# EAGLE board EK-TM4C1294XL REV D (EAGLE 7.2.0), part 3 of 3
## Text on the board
Bottom: EK-TM4C1294XL / REV D
tPlace: DEBUG | TXD | RXD | Target USB | TCK | TMS | TDI | BoosterPack 2 | TDO | BoosterPack 1 | !RESET | TM | Tiva C Series / Connected LaunchPad | 85 | 71 | 57 | 43 | 29 | 15 | 1
bPlace: TXD | RXD | TCK | TMS | TDI | TDO | !RESET
tNames: POWER | http://www.ti.com/launchpad | POWER SELECT | U22 | BoosterPack | +3v3 | OTG | ICDI | U14 | CAN | UART | MCU 3V3 | Y2 | CAN | Y1 | UART | EK-TM4C1294XL Rev D
bNames: +3v3 / PD2 / PP0 / PP1 / See JP4 / See JP5 / PQ0 / PP4 / PN5 / PN4 | +5V / GND / PB4 / PB5 / PK0 / PK1 / PK2 / PK3 / PA4 / PA5 | TP1 | TP8 | +3V3 / PE4 / PC4 / PC5 / PC6 / PE5 / PD3 / PC7 / PB2 / PB3 | TP10 | TP13 | TP3 | +5V / GND / PE0 / PE1 / PE2 / PE3 / PD7 / PA6 / PM4 / PM5 | TP9 | BP2_A2.6 / PA1 | PD5 / ICDI_TX | TP4 | TP5 | PG1 / PK4 / PK5 / PM0 / PM1 / PM2 / PH0 / PH1 / PK6 / PK7 | TP12 | BP2_A2.5 / PA0 | PD4 / ICDI RX | TP2 | TP6 | TP11 | PF1 / PF2 / PF3 / PG0 / PL4 / PL5 / PL0 / PL1 / PL2 / PL3 | TP7 | GND / PM7 / PP5 / PA7 / !RESET / PQ2/PA3 / PQ3/PA2 / PP3 / PQ1 / PM6 | GND / PM3 / PH2 / PH3 / !RST / PD1 / PD0 / PN2 / PN3 / PP2 | 5V / 3V3 | !WAK / GND | PQ4 / !RST | PN3 / PM4 | PN2 / PM5 | PN1 / PM6 | PN0 / PM7 | PN5 / PJ1 | PN4 / PJ0 | PL5 / PP5 | PK4 / PP4 | PK5 / PA1 | PP3 / PA0 | PP2 / PF3 | PB3 / PF2 | PB2 / PF1 | PL4 / PF0 | PK6 / PF4 | GND / GND | PK7 / PB1 | PQ3 / PB0 | PQ2 / PP1 | PQ1 / PP0 | PQ0 / PD2 | PL3 / PD0 | PL2 / PD1 | PL1 / PD3 | PL0 / PD6 | PM0 / PD7 | PM1 / PD4 | PM2 / PD5 | GND / GND | PM3 / REF | PG0 / PK3 | PG1 / PK2 | PA7 / PK1 | PA6 / PK0 | PC4 / PE5 | PC5 / PE4 | PC6 / PE3 | PC7 / PE2 | PH3 / PE1 | PH2 / PE0 | PH1 / PA5 | PH0 / PA4 | PB5 / PA3 | PB4 / PA2 | GND / GND | 3V3 / 5V
Document: Layer Stackup / Top silkscreen / Top Solder Mask / Component Side / Layer 2 / Layer 3 / Solder Side / Bottom Solder Mask / Bottom Silkscreen | File Names / EK-TM4C129EXL.sst / EK-TM4C129EXL.smt / EK-TM4C129EXL.l1 / EK-TM4C129EXL.l2 / EK-TM4C129EXL.l3 / EK-TM4C129EXL.l4 / EK-TM4C129EXL.smb / EK-TM4C129EXL.ssb | NOTES: UNLESS OTHERWISE SPECIFIED / 1) Manufacture in accordance with IPC-6012, Type 3, Class 2. / 2) End Product Features shall not vary more than 20% from artwork originals / 3) Material shall be ROHS compliant, copper clad FR-406, NEMA Grade (Tg 170degC) / Per IPC-4101, Color Natural, or equivalent / 4) Construction shall be symetrical multilayer per layer stackup detail / 5) Copper weight on inner layers shall be 1 oz per square foot / 6) Equivalent copper weight on outler layers shall be 1.0 oz per square foot before plating / 7) All plated through holes shall have a minimum of 0.0007 inches of copper / 8) Drill hole tolerance after plating shall be +/- 0.003 inches / 9) Minimum annular ring shall be 0.001 inches / 10) Minmum annular rint at emergent conductors shall be 0.003 inches / 11) PCB Thickness shall be 0.062 inches +/- 0.007 inches / 12) Warp / Twist shall not exceed 0.010 inches per inch / 13) Finish shall be LPI, Gloss RED SMOBC, Both sides balance of exposed copper shall be HASL / 14) Silkscreen with nonconductive white epoxy ink / 15) Board stack-up should be targetted such that a differential impedance of 90 ohms +/- 10% can / be achieved on the top layer with 10.8 mil traces and 6 mil spacing. Additionally 100 ohm +/- 10% / with 8.7 mil traces and 6 mil spacing. Boards do not need to be impedance controlled.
